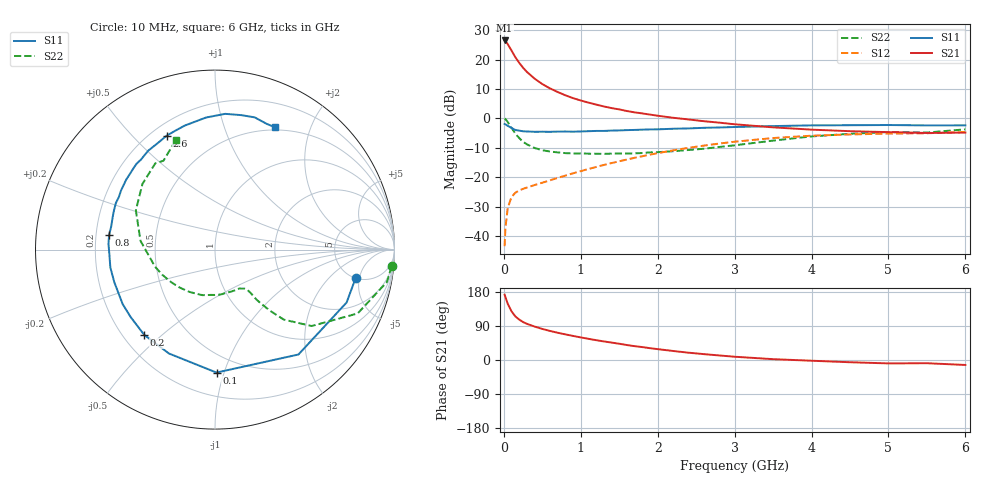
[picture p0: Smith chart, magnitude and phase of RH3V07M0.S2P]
! SIEMENS Small Signal Semiconductors
! BFR106
! Si NPN RF Bipolar Junction Transistor in SOT23
! VCE = 3 V  IC = 7 mA
! Common Emitter S-Parameters:  August  1996
# GHz  S  MA  R  50
!  f  S11  S21  S12  S22
! GHz  MAG  ANG  MAG  ANG  MAG  ANG  MAG  ANG
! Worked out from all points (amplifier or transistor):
!   36 points, 10 MHz to 6 GHz, reference 50 ohm
!   highest |S21| = 26.5 dB at 10 MHz (marker M1)
!   |S21| within 3 dB of that: start of sweep to 90.11 MHz
!   unconditionally stable (mu >= 1): 549.9 MHz to 2.117 GHz; 4.842 GHz to end of sweep
!   at 250 MHz: K = 0.60, MSG = 20.6 dB, |S12| = -24.0 dB
!   at 1.4 GHz: K = 1.13, MAG = 7.2 dB, |S12| = -15.2 dB
!   at 6 GHz: K = 1.02, MAG = -0.9 dB, |S12| = -4.6 dB
!   S11 on the Smith chart (normalised r, x): 10 MHz: 5.03, -4.41; 100 MHz: 0.37, -0.94; 200 MHz: 0.29, -0.44; 800 MHz: 0.25, +0.06; 2.6 GHz: 0.26, +0.63; 6 GHz: 0.47, +1.50
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0.01  0.7995 -11.4  21.08 172.4  0.0067 85.3  0.9885 -5.4
0.02  0.7903 -21.9  20.65 166.5  0.0133 78.2  0.9744 -10.7
0.05  0.7468 -51.5  18.28 148.6  0.0297 64.9  0.8709 -24.1
0.1  0.6852 -89.3  14.19 128.4  0.0462 51.4  0.687 -38.3
0.15  0.6332 -113.9  10.9 114.9  0.0543 44.2  0.547 -45.5
0.2  0.6174 -129.7  8.781 106.7  0.0595 41.8  0.4619 -47.9
0.25  0.6017 -141.3  7.234 100.1  0.0632 41.1  0.3985 -49.5
0.3  0.5975 -149.4  6.143 95.5  0.0666 41.9  0.3616 -50.3
0.4  0.5897 -162.0  4.727 88.2  0.0734 44.1  0.3127 -50.6
0.5  0.5915 -170.3  3.821 82.0  0.0804 46.9  0.2868 -51.2
0.6  0.5892 -177.6  3.226 76.7  0.0883 49.8  0.2723 -53.0
0.8  0.5958 172.2  2.462 67.6  0.1061 54.0  0.2559 -58.1
0.9  0.5924 167.5  2.202 63.5  0.1162 55.8  0.2528 -60.7
1.1  0.6039 158.7  1.849 55.9  0.1374 58.0  0.2507 -68.4
1.3  0.6103 151.4  1.591 49.0  0.161 59.2  0.2488 -76.5
1.6  0.63 141.7  1.329 39.5  0.1991 59.0  0.2527 -90.5
2.2  0.6648 124.1  1.021 23.8  0.2851 54.2  0.2755 -121.3
2.6  0.6895 113.0  0.893 15.5  0.3435 48.6  0.304 -143.2
3.5  0.7375 93.9  0.702 2.2  0.4621 33.1  0.418 173.3
4.5  0.7634 78.9  0.604 -5.9  0.5321 15.1  0.5453 137.8
5.5  0.7576 67.7  0.563 -8.5  0.5577 4.1  0.5723 120.1
6  0.7591 63.9  0.572 -13.1  0.5856 -3.6  0.65 109.5
